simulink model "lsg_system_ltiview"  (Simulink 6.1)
settings: Solver=ode45  StartTime=0.0  StopTime=Tstop  MaxStep=max_step  RelTol=1e-3
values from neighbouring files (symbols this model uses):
  den = [0.02 1]    [lsg_regelung_ini.m]    (also in lsg_system_ini.m; lsg_sys_kalman_ini.m; system_ini.m; sys_kalman_ini.m)
  g = 2    [lsg_regelung_ini.m]    (also in lsg_system_ini.m; lsg_sys_kalman_ini.m; system_ini.m; sys_kalman_ini.m)
  num = 2    [lsg_regelung_ini.m]    (also in lsg_system_ini.m; lsg_sys_kalman_ini.m; system_ini.m; sys_kalman_ini.m)
  p = [-2 -3+10*i -3-10*i]    [lsg_regelung_ini.m]    (also in lsg_system_ini.m; lsg_sys_kalman_ini.m; system_ini.m; sys_kalman_ini.m)
  verst = 100    [lsg_regelung_ini.m]    (also in lsg_system_ini.m; lsg_sys_kalman_ini.m; system_ini.m; sys_kalman_ini.m)
  z = [1 1]    [lsg_regelung_ini.m]    (also in lsg_system_ini.m; lsg_sys_kalman_ini.m; system_ini.m; sys_kalman_ini.m)

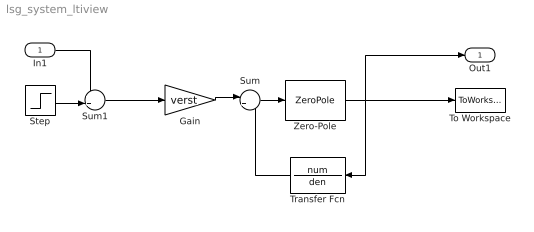
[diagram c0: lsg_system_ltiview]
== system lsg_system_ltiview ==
  In1 : Inport  Port=1  LatchInput=off
  Gain : Gain  Gain=verst
  Step : Step  Time=0  SampleTime=0
  Sum : Sum  Inputs=|++
  Sum1 : Sum  Inputs=++|
  To Workspace : ToWorkspace  VariableName=y  SampleTime=-1  SaveFormat=Array
  Transfer Fcn : TransferFcn  Orientation=left  Numerator=num  Denominator=den
  Zero-Pole : ZeroPole  Zeros=z  Poles=p  Gain=g
  Out1 : Outport
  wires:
  Zero-Pole/1 -> Transfer Fcn/1, Out1/1, To Workspace/1
  Transfer Fcn/1 -> Sum/2
  Sum/1 -> Zero-Pole/1
  Gain/1 -> Sum/1
  Step/1 -> Sum1/2
  In1/1 -> Sum1/1
  Sum1/1 -> Gain/1
